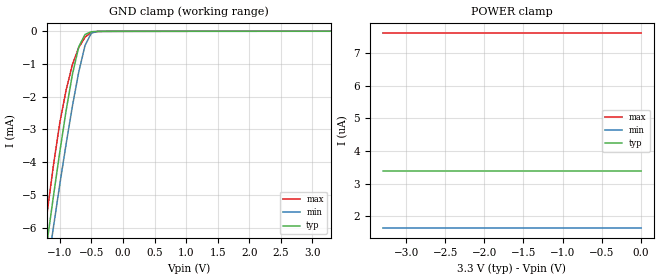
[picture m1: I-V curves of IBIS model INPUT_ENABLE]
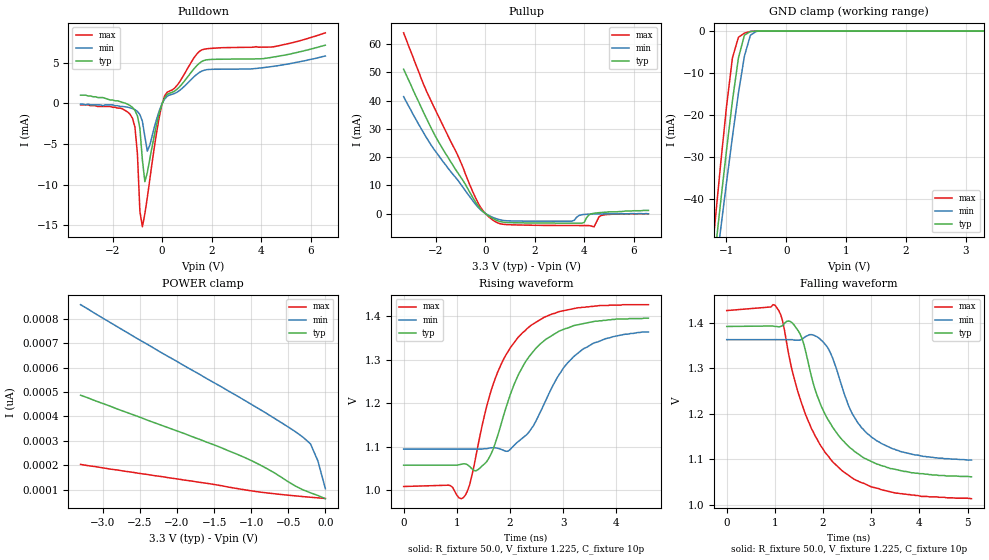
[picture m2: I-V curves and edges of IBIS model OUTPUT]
|   Texas Instruments Incorporated
|   Data Transmissions Products
|   IBIS Model for SN65LVDS047
|   16D SOIC Package
[IBIS Ver]   3.2
[Comment char]   |_char
[File name]   lvds047d.ibs
[File Rev]   1.0
[Date]   22Aug00
[Source]   File originated at Texas Instruments Incorporated.
   Data Transmission Products Group.
[Notes]
[Disclaimer]
(C) Copyright Texas Instruments Incorporated 2000
   All rights reserved
  Texas Instruments Incorporated hereby grants the user of this IBIS
model a non-exclusive, nontransferable license to use this IBIS model
under the following terms.  Before using this IBIS model, the user
should read this license.  If the user does not accept these terms,
the IBIS model should be returned to Texas Instruments within 30 days.
  The user is granted this license only to use the IBIS model and
is not granted rights to sell, load, rent, lease or license the IBIS
model in whole or in part, or in modified form to anyone other than
user.  User may modify the IBIS model to suit its specific applications
but rights to derivative works and such modifications shall belong to
Texas Instruments.
  This IBIS model is provided on an "AS IS" basis and Texas Instruments
makes absolutely no warranty with respect to the information contained
herein.  TEXAS INSTRUMENTS DISCLAIMS AND CUSTOMER WAIVES ALL WARRANTIES,
EXPRESS OR IMPLIED, INCLUDING WARRANTIES OF MERCHANTABILITY OR FITNESS
FOR A PARTICULAR PURPOSE. The entire risk as to quality and performance
is with the Customer. ACCORDINGLY, IN NO EVENT SHALL THE COMPANY BE LIABLE
FOR ANY DAMAGES, WHETHER IN CONTRACT OR TORT,INCLUDING ANY LOST PROFITS
OR OTHER INCIDENTAL, CONSEQUENTIAL, EXEMPLARY, OR PUNITIVE DAMAGES ARISING
OUT OF THE USE OR APPLICATION OF THE IBIS model provided in this package.
Further, Texas Instruments reserves the right to discontinue or make changes
without notice to any product herein to improve reliability, function, or
design. Texas Instruments does not convey any license under patent rights
or any other intellectual property rights, including those of third parties.
Contact Texas Instruments at ATTN:DATA TRANSMISSIONS
[Copyright]   Copyright 2000, Texas Instruments, All Rights Reserved
[Component]   LVDS047D
[Manufacturer]  Texas Instruments Incorporated
[Package]
|   typ   min   max
R_pkg   0.035   0.030   0.040
L_pkg   2.181nH   1.231nH   3.257nH
C_pkg   0.322pF   0.163pF   0.546pF
[Pin]   signal_name   model_name   R_pin   L_pin   C_pin
1   EN   INPUT_ENABLE   0.040   3.251n   0.546p
2   DIN1   INPUT_ENABLE   0.039   2.561n   0.393p
3   DIN2   INPUT_ENABLE   0.030   1.681n   0.186p
4   VCC   POWER   0.030   1.231n   0.163p
5   GND   GND   0.030   1.231n   0.163p
6   DIN3   INPUT_ENABLE   0.030   1.681n   0.186p
7   DIN4   INPUT_ENABLE   0.039   2.564n   0.393p
8   /EN   INPUT_ENABLE   0.040   3.257n   0.545p
9   DOUT4-   OUTPUT   0.040   3.247n   0.546p
10   DOUT4+   OUTPUT   0.039   2.558n   0.394p
11   DOUT3-   OUTPUT   0.030   1.681n   0.187p
12   DOUT3+   OUTPUT   0.030   1.231n   0.163p
13   DOUT2-   OUTPUT   0.030   1.231n   0.163p
14   DOUT2+   OUTPUT   0.030   1.681n   0.187p
15   DOUT1-   OUTPUT   0.039   2.558n   0.394p
16   DOUT1+   OUTPUT   0.040   3.246n   0.546p
[Diff_pin]   inv_pin   vdiff   tdelay_typ   tdelay_min   tdelay_max
| The 'xY' pin is Diff_pin and the 'xZ' pin is the inv_pin
16   15   NA   0 0 0
14   13   NA   0 0 0
12   11   NA   0 0 0
10   9   NA   0 0 0
| Models and submodels in the file (2): INPUT_ENABLE (Input), OUTPUT (3-state)
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|   Driver Input / Enable Model
[Model]   INPUT_ENABLE
Model_type   Input
|Signals   EN,/EN,DIN1,DIN2,DIN3,DIN4
Vinh = 2.0
Vinl = 0.8
|   typ   min   max
C_comp   1.10pF   1.02pF   1.21pF
|   typ   min   max
[Temperature Range]   25.0   -40   85
[Voltage range]   3.3V   3.0V   3.6V
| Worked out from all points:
|   GND clamp passes 1 mA (typ) near -0.76 V on its own axis
[GND_clamp]
|Voltage  I(typ)   I(min)   I(max)
-3.3V     -42.9mA    -42.4mA    -44.1mA
-1.3V     -7.87mA    -8.69mA    -7.06mA
-1.2V     -6.42mA    -7.31mA    -5.53mA
-1.1V     -5.02mA    -5.97mA    -4.08mA
-1V       -3.68mA    -4.67mA    -2.79mA
-900mV    -2.42mA    -3.44mA    -1.79mA
-800mV    -1.31mA    -2.28mA    -1.01mA
-700mV    -472uA     -1.24mA    -495uA
-600mV    -93.4uA    -429uA     -177uA
-500mV    -12.6uA    -53.4uA    -28.7uA
-400mV    -2.23uA    -3.52uA    -4.22uA
3.3V      3.38uA     1.63uA     7.62uA
[Power_clamp]
| Note that the[POWER_clamp]voltage table is referenced to Vcc
| and is calculated using Vtable=Vcc - Vmeasured.
|Voltage  I(typ)   I(min)   I(max)
-3.3V     3.38uA     1.63uA     7.62uA
-3.2V     3.38uA     1.63uA     7.62uA
-3.1V     3.38uA     1.63uA     7.62uA
0V        3.38uA     1.63uA     7.62uA
|   Driver Output Model
[Model]   OUTPUT
Model_type   3-state
| Signals   DOUT1+,DOUT1-,DOUT2+,DOUT2-,DOUT3+,DOUT3-,DOUT4+,DOUT4-
Vmeas = 1.2V   |Reference voltage for timing measurements
Cref = 10pF   |Timing specification test load capacitance value
Rref = 50   |Note: 50 Ohm load; single ended configuration
Vref = 1.20V   |Timing specification test load voltage
| variable   typ   min   max
C_comp   3.66pF   3.56pF   3.92pF
|   typ   min   max
[Temperature Range]   25.0   -40   85
[Voltage range]   3.3V   3.0V   3.6V
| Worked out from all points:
|   slope of the pulldown table from 0 to 0.495 V, typ, clamps not added: 326 ohm
|   slope of the pullup table from 0 to 0.495 V, typ, clamps not added: 192 ohm
|   GND clamp passes 1 mA (typ) near -0.70 V on its own axis
|   rising waveform, R_fixture 50.0, V_fixture 1.225, C_fixture 10p: 20-80 % time 733ps typ, 783ps min, 719ps max; typ from 1.06 V to 1.4 V
|   falling waveform, R_fixture 50.0, V_fixture 1.225, C_fixture 10p: 20-80 % time 875ps typ, 740ps min, 923ps max; typ from 1.39 V to 1.06 V
[Pulldown]
|Voltage  I(typ)   I(min)   I(max)
-3.3V     1mA        -100uA     -200uA
-1.7V     200uA      -400uA     -600uA
-1.2V     -520uA     -650uA     -1.85mA
-1.1V     -880uA     -790uA     -2.94mA
-1V       -1.55mA    -1.01mA    -6.24mA
-900mV    -3.1mA     -1.4mA     -13.3mA
-800mV    -6.95mA    -2.21mA    -15.2mA
-700mV    -9.64mA    -4.09mA    -13.6mA
-600mV    -8.52mA    -5.89mA    -11.6mA
0V        -34.7uA    -30.8uA    -40.1uA
1.4V      4.62mA     3.55mA     6.05mA
6.6V      7.14mA     5.81mA     8.66mA
[Pullup]
| Note that the[Pullup]voltage table is referenced to Vcc
| and is calculated using Vtable=Vcc - Vmeasured.
|Voltage  I(typ)   I(min)   I(max)
-3.3V     51.1mA     41.4mA     64mA
-2.4V     34.1mA     27.2mA     43.8mA
-1.7V     22.6mA     18.3mA     31mA
-1.1V     14.3mA     11.7mA     20.4mA
-300mV    2.89mA     2.33mA     3.94mA
300mV     -1.72mA    -1.33mA    -2.27mA
800mV     -3.13mA    -2.51mA    -3.87mA
3.5V      -3.4mA     -2.71mA    -4.24mA
3.9V      -3.4mA     -430uA     -4.25mA
4.4V      110uA      -160uA     -4.71mA
4.7V      370uA      -200uA     -670uA
6.6V      1.1mA      -100uA     -100uA
[GND_clamp]
| Outputs in High Impedance (off)
|Voltage  I(typ)   I(min)   I(max)
-3.3V     -347mA     -323mA     -383mA
-1.3V     -67.3mA    -71.1mA    -62mA
-1.2V     -54.1mA    -59.3mA    -46.9mA
-1.1V     -41.1mA    -47.6mA    -32.1mA
-1V       -28.5mA    -36.2mA    -18.1mA
-900mV    -16.6mA    -25.2mA    -6.38mA
-800mV    -6.42mA    -14.8mA    -1.5mA
-700mV    -997uA     -5.97mA    -506uA
-600mV    -101uA     -992uA     -108uA
-500mV    -8.6uA     -72.8uA    -9.14uA
3.3V      64pA       315pA      54.2pA
[POWER_clamp]
| Note that the [POWER_clamp] voltage table is referenced to Vcc
| and is calculated using Vtable = Vcc - Vmeasured.
| Outputs in Tri-state.
|Voltage  I(typ)   I(min)   I(max)
-3.3V     487pA      857pA      204pA
-2.5V     397pA      712pA      167pA
-1.5V     284pA      538pA      122pA
-1.2V     247pA      486pA      106pA
-800mV    189pA      414pA      88pA
-400mV    115pA      337pA      75.3pA
-300mV    100pA      315pA      72.5pA
-200mV    88pA       288pA      69.8pA
-100mV    77pA       218pA      67.4pA
0V        64pA       105pA      64.9pA
[Ramp]
|   Simulation with 100 ohm and 10pF loads.
|   typ   min   max
dV/dt_r   0.200/711ps   0.161/777ps   0.249/712ps
dV/dt_f   0.200/897ps   0.160/760ps   0.250/945ps
R_load = 50ohm
[Rising Waveform]
R_fixture = 50.0
V_fixture = 1.225
V_fixture_min = 1.229
V_fixture_max = 1.218
C_fixture = 10p
L_fixture = 0n
|   V(typ)  V(min)  V(max)
0s        1.058V     1.095V     1.009V
840ps     1.058V     1.095V     1.012V
1.16ns    1.061V     1.095V     989mV
1.44ns    1.052V     1.095V     1.129V
1.76ns    1.123V     1.097V     1.27V
2.08ns    1.245V     1.104V     1.34V
2.4ns     1.314V     1.142V     1.38V
3.2ns     1.379V     1.308V     1.418V
3.8ns     1.391V     1.349V     1.425V
4.6ns     1.396V     1.364V     1.427V
[Falling Waveform]
R_fixture = 50.0
V_fixture = 1.225
V_fixture_min = 1.229
V_fixture_max = 1.218
C_fixture = 10p
L_fixture = 0n
|   V(typ)  V(min)  V(max)
0s        1.392V     1.363V     1.427V
1ns       1.392V     1.363V     1.439V
1.16ns    1.394V     1.363V     1.404V
1.32ns    1.403V     1.363V     1.313V
1.52ns    1.376V     1.362V     1.234V
2ns       1.208V     1.358V     1.122V
2.4ns     1.142V     1.257V     1.074V
2.72ns    1.112V     1.18V      1.052V
3.2ns     1.086V     1.135V     1.033V
5.08ns    1.061V     1.098V     1.013V
